| IBIS file k60_2m_180mhz_144mapbga_13x13_xn73j_derated.ibs generated by Viper version: 2018.10.16
[IBIS Ver]   4.2
[Comment Char]   |_char
[File Name]   k60_2m_180mhz_144mapbga_13x13_xn73j_derated.ibs
[File Rev]   1.0
[Date]   Tue Oct 16 17:54:02 2018
[Source]   NXP Viper 2018.10.16
[Notes]
[Disclaimer] IMPORTANT NOTICE
  This information is provided on an AS IS basis and without warranty.
  IN NO EVENT SHALL NXP BE LIABLE FOR INCIDENTAL OR CONSEQUENTIAL
  DAMAGES ARISING FROM USE OF THIS INFORMATION. THIS DISCLAIMER OF
  WARRANTY EXTENDS TO THE USER OF THE INFORMATION, AND TO THEIR CUSTOMERS
  OR USERS OF PRODUCTS  AND IS IN LIEU OF ALL WARRANTIES WHETHER EXPRESS,
  IMPLIED, OR STATUTORY, INCLUDING IMPLIED WARRANTIES OF MERCHANTABILITY
  OR FITNESS FOR PARTICULAR PURPOSE.
  NXP does not represent or warrant that the information furnished
  hereunder is free of infringement of any third party patents,
  copyrights, trade secrets, or other intellectual property rights.
  NXP does not represent or warrant that the information is free of
  defect, or that it meets any particular standard, requirements or need
  of the user of the infomation or their customers.
  NXP reserves the right to change the information in this file
  without notice.
   http://www.nxp.com
[Copyright]   (C) Copyright NXP 2004 - 2018, All Rights Reserved.
|   k60_2m_144mapbga_13x13
[Component]   k60_2m_144mapbga_13x13
[Manufacturer]   NXP
[Package]
| variable   typ   min   max
R_pkg   0.13037   0.042059   0.28237
L_pkg   2.200e-09   1.007e-09   4.756e-09
C_pkg   1.108e-12   8.202e-13   2.263e-12
[Pin] signal_name   model_name   R_pin   L_pin   C_pin
A1   PTD7   p_io_fast_hd_84u3v_6m   0.1767   3.230e-09 1.380e-12
A2   PTD6   p_io_fast_hd_84u3v_6m   0.24124   3.607e-09 1.256e-12
A3   PTD5   p_io_fast_hd_84u3v_6m   0.20685   3.225e-09 1.178e-12
A4   PTD4   p_io_fast_hd_84u3v_6m   0.1989   3.110e-09 1.168e-12
A5   PTD0   p_io_fast_84u3v_6m   0.16563   2.686e-09 1.012e-12
A6   PTC16   p_io_fast_84u3v_6m   0.16815   2.638e-09 1.005e-12
A7   PTC12   p_io_fast_84u3v_6m   0.15584   2.576e-09 1.008e-12
A8   PTC8   p_io_fast_84u3v_6m   0.15772   2.632e-09 9.509e-13
A9   PTC4   p_io_fast_hd_84u3v_6m   0.12744   2.310e-09 9.538e-13
A11   PTC3   p_io_fast_hd_84u3v_6m   0.17723   2.897e-09 1.109e-12
A12   PTC2   p_io_fast_84u3v_6m   0.20689   3.392e-09 1.147e-12
B1   PTD12   p_io_fast_84u3v_6m   0.20681   3.347e-09 1.070e-12
B2   PTD11   p_io_fast_84u3v_6m   0.15374   2.624e-09 1.135e-12
B3   PTD10   p_io_fast_84u3v_6m   0.14183   2.420e-09 1.169e-12
B4   PTD3   p_io_fast_84u3v_6m   0.15752   2.572e-09 1.158e-12
B5   PTC19   p_io_fast_84u3v_6m   0.14305   2.368e-09 9.679e-13
B6   PTC15   p_io_fast_84u3v_6m   0.18186   2.838e-09 1.206e-12
B7   PTC11   p_io_fast_84u3v_6m   0.1211   2.128e-09 1.062e-12
B8   PTC7   p_io_fast_84u3v_6m   0.115   2.073e-09 9.642e-13
B9   PTD9   p_io_fast_84u3v_6m   0.28237   4.756e-09 2.263e-12
B11   PTC1   p_io_fast_84u3v_6m   0.15165   2.581e-09 1.116e-12
B12   PTC0   p_io_fast_84u3v_6m   0.17659   2.976e-09 1.058e-12
C1   PTD15   p_io_fast_84u3v_6m   0.1459   2.559e-09 1.032e-12
C2   PTD14   p_io_fast_84u3v_6m   0.11803   2.152e-09 9.752e-13
C3   PTD13   p_io_fast_84u3v_6m   0.10442   1.941e-09 1.039e-12
C4   PTD2   p_io_fast_84u3v_6m   0.1542   2.591e-09 1.174e-12
C5   PTC18   p_io_fast_84u3v_6m   0.13918   2.329e-09 1.232e-12
C6   PTC14   p_io_fast_84u3v_6m   0.14045   2.324e-09 1.243e-12
C7   PTC10   p_io_fast_84u3v_6m   0.091438  1.815e-09 1.163e-12
C8   PTC6   p_io_fast_84u3v_6m   0.095955  1.862e-09 1.095e-12
C9   PTD8   p_io_fast_84u3v_6m   0.17703   3.145e-09 1.523e-12
C11   PTB23   p_io_fast_84u3v_6m   0.12401   2.224e-09 1.010e-12
C12   PTB22   p_io_fast_84u3v_6m   0.16109   2.737e-09 1.000e-12
D1   PTE2   p_io_fast_84u3v_6m   0.15458   2.571e-09 9.707e-13
D2   PTE1   p_io_fast_84u3v_6m   0.084672  1.697e-09 9.052e-13
D3   PTE0   p_io_fast_84u3v_6m   0.080898  1.614e-09 9.614e-13
D4   PTD1   p_io_fast_84u3v_6m   0.1196   2.013e-09 1.284e-12
D5   PTC17   p_io_fast_84u3v_6m   0.11589   1.937e-09 1.329e-12
D6   PTC13   p_io_fast_84u3v_6m   0.12216   2.016e-09 1.294e-12
D7   PTC9   p_io_fast_84u3v_6m   0.10769   1.891e-09 1.275e-12
D8   PTC5   p_io_fast_84u3v_6m   0.083046  1.529e-09 1.075e-12
D9   PTB21   p_io_fast_84u3v_6m   0.069786  1.388e-09 1.081e-12
D10   PTB20   p_io_fast_84u3v_6m   0.072983  1.512e-09 1.080e-12
D11   PTB19   p_io_fast_84u3v_6m   0.11729   2.101e-09 1.049e-12
D12   PTB18   p_io_fast_84u3v_6m   0.15379   2.582e-09 9.778e-13
E1   PTE6   p_io_fast_84u3v_6m   0.15201   2.497e-09 9.728e-13
E2   PTE5   p_io_fast_84u3v_6m   0.072065  1.467e-09 9.777e-13
E3   PTE4   p_io_fast_84u3v_6m   0.15445   2.567e-09 1.210e-12
E4   PTE3   p_io_fast_84u3v_6m   0.091528  1.512e-09 1.079e-12
E5   VDD   POWER   NA   NA   NA
E6   VDD   POWER   NA   NA   NA
E7   VDD   POWER   NA   NA   NA
E8   VDD   POWER   NA   NA   NA
E9   PTB17   p_io_fast_84u3v_6m   0.090018  1.530e-09 1.105e-12
E10   PTB16   p_io_fast_84u3v_6m   0.071785  1.356e-09 1.033e-12
E11   PTB11   p_io_fast_84u3v_6m   0.1174   2.042e-09 9.782e-13
E12   PTB10   p_io_fast_84u3v_6m   0.14971   2.513e-09 1.021e-12
F1   PTE10   p_io_fast_84u3v_6m   0.1489   2.421e-09 9.276e-13
F2   PTE9   p_io_fast_84u3v_6m   0.11513   1.993e-09 1.042e-12
F3   PTE8   p_io_fast_84u3v_6m   0.15002   2.498e-09 1.179e-12
F4   PTE7   p_io_fast_84u3v_6m   0.086683  1.500e-09 1.160e-12
F5   VDD   POWER   NA   NA   NA
F6   VSS   GND   NA   NA   NA
F7   VSS   GND   NA   NA   NA
F8   VDD   POWER   NA   NA   NA
F9   PTB9   p_io_fast_84u3v_6m   0.059202  1.173e-09 1.018e-12
F10   PTB8   p_io_fast_84u3v_6m   0.070195  1.393e-09 9.710e-13
F11   PTB7   p_io_fast_84u3v_6m   0.10803   1.929e-09 9.562e-13
F12   PTB6   p_io_fast_84u3v_6m   0.14447   2.427e-09 9.618e-13
G1   VREGOUT   POWER   0.063206  1.451e-09 1.324e-12
G2   VREGIN0   POWER   0.042059  1.007e-09 1.354e-12
G3   PTE12   p_io_fast_84u3v_6m   0.075407  1.340e-09 1.180e-12
G4   PTE11   p_io_fast_84u3v_6m   0.080602  1.557e-09 1.230e-12
G5   VREFH   POWER   NA   NA   NA
G6   VREFL   NC   NA   NA   NA
G7   VSS   GND   NA   NA   NA
G8   VSS   GND   NA   NA   NA
G9   PTB5   p_io_fast_84u3v_6m   0.08967   1.495e-09 1.046e-12
G10   PTB4   p_io_fast_84u3v_6m   0.067218  1.294e-09 9.258e-13
G11   PTB3   p_io_fast_84u3v_6m   0.11289   1.909e-09 9.538e-13
G12   PTB2   p_io_fast_84u3v_6m   0.15155   2.485e-09 9.892e-13
H1   USB0DP   NC   0.17782   2.688e-09 1.062e-12
H2   USB0DM   NC   0.16924   2.555e-09 1.175e-12
H3   VSS   GND   NA   NA   NA
H4   PTE28   p_io_fast_84u3v_6m   0.13628   2.231e-09 1.535e-12
H5   VDDA   POWER   NA   NA   NA
H6   VSSA   GND   NA   NA   NA
H7   VSS   GND   NA   NA   NA
H8   VSS   GND   NA   NA   NA
H9   PTB1   p_io_fast_hd_84u3v_6m   0.088545  1.541e-09 1.078e-12
H10   PTB0   p_io_fast_hd_84u3v_6m   0.07193   1.458e-09 1.011e-12
H11   PTA29   p_io_fast_84u3v_6m   0.1092   1.928e-09 9.740e-13
H12   PTA28   p_io_fast_84u3v_6m   0.1489   2.462e-09 9.911e-13
J1   USB1DP   NC   0.15803   2.269e-09 9.367e-13
J2   VREGIN1   POWER   0.068056  1.347e-09 1.170e-12
J3   ADC0SE16_CMP1IN2_ADC0SE21   NC   0.08836   1.703e-09 1.177e-12
J4   PTE27   p_io_fast_84u3v_6m   0.13178   2.323e-09 1.598e-12
J5   PTA0   p_io_fast_84u3v_6m   0.153   2.517e-09 1.320e-12
J6   PTA1   p_io_fast_84u3v_6m   0.13311   2.225e-09 1.256e-12
J7   PTA6   p_io_fast_84u3v_6m   0.062001  1.109e-09 1.055e-12
J8   PTA7   p_io_fast_84u3v_6m   0.084534  1.447e-09 1.157e-12
J9   PTA13   p_io_fast_84u3v_6m   0.07581   1.411e-09 1.087e-12
J10   PTA27   p_io_fast_84u3v_6m   0.062053  1.319e-09 1.092e-12
J11   PTA26   p_io_fast_84u3v_6m   0.109   1.945e-09 9.549e-13
J12   PTA25   p_io_fast_84u3v_6m   0.14712   2.455e-09 9.664e-13
K1   USB1DM   NC   0.15596   2.273e-09 9.297e-13
K2   VSS   GND   NA   NA   NA
K3   ADC1SE16_CMP2IN2_ADC0SE22   NC   0.093833  1.575e-09 9.911e-13
K4   PTE26   p_io_fast_84u3v_6m   0.11535   2.135e-09 1.578e-12
K5   PTE25   p_io_fast_84u3v_6m   0.071914  1.400e-09 1.592e-12
K6   PTA2   p_io_fast_84u3v_6m   0.075006  1.515e-09 1.067e-12
K7   PTA3   p_io_fast_84u3v_6m   0.076031  1.521e-09 9.091e-13
K8   PTA8   p_io_fast_84u3v_6m   0.16395   2.596e-09 1.171e-12
K9   PTA12   p_io_fast_84u3v_6m   0.077963  1.574e-09 1.040e-12
K10   PTA16   p_io_fast_84u3v_6m   0.12551   2.032e-09 1.168e-12
K11   PTA17   p_io_fast_84u3v_6m   0.14656   2.272e-09 1.166e-12
K12   PTA24   p_io_fast_84u3v_6m   0.12128   2.134e-09 9.407e-13
L1   USB1VBUS   POWER   0.090888  1.827e-09 1.559e-12
L2   ADC0DM0_ADC1DM3   NC   0.18325   2.692e-09 1.086e-12
L3   DAC0OUT_CMP1IN3_ADC0SE23   NC   0.11875   2.000e-09 8.994e-13
L4   DAC1OUT_CMP0IN4_CMP2IN3_ADC1SE23   NC   0.11014   1.898e-09 9.220e-13
L5   TAMPER0   p_io_84u3v_6m   0.12121   2.052e-09 1.037e-12
L6   VBAT   POWER   NA   NA   NA
L7   PTA4   p_io_flt_84u3v_6m   0.11174   1.932e-09 9.675e-13
L8   PTA9   p_io_fast_84u3v_6m   0.11121   1.866e-09 9.390e-13
L9   PTA11   p_io_fast_84u3v_6m   0.12511   2.024e-09 1.052e-12
L10   PTA14   p_io_fast_84u3v_6m   0.14162   2.139e-09 1.035e-12
L11   PTA15   p_io_fast_84u3v_6m   0.15537   2.405e-09 1.085e-12
L12   RESETB   p_vpp_84u3v_6m   0.12232   2.220e-09 1.068e-12
M1   ADC1DP0_ADC0DP3   NC   0.22009   3.293e-09 1.235e-12
M2   ADC1DM0_ADC0DM3   NC   0.22652   3.293e-09 1.206e-12
M3   VREFOUT_CMP1IN5_CMP0IN5_ADC1SE18   NC   0.17041   2.710e-09 9.453e-13
M4   PTE24   p_io_fast_84u3v_6m   0.18414   2.868e-09 1.024e-12
M6   EXTAL32   NC   0.13257   2.260e-09 8.202e-13
M7   XTAL32   NC   0.18902   3.006e-09 1.031e-12
M8   PTA5   p_io_fast_84u3v_6m   0.1639   2.449e-09 1.034e-12
M9   PTA10   p_io_fast_84u3v_6m   0.16013   2.533e-09 1.014e-12
M10   VSS   GND   NA   NA   NA
M11   PTA19   p_io_fast_84u3v_6m   0.21862   3.056e-09 1.159e-12
M12   PTA18   p_io_fast_84u3v_6m   0.17651   2.672e-09 1.041e-12
[Pin Mapping]   pulldown_ref   pullup_ref
A1   NC   NC
A2   NC   NC
A3   NC   NC
A4   NC   NC
A5   NC   NC
A6   NC   NC
A7   NC   NC
A8   NC   NC
A9   NC   NC
A11   NC   NC
A12   NC   NC
B1   NC   NC
B2   NC   NC
B3   NC   NC
B4   NC   NC
B5   NC   NC
B6   NC   NC
B7   NC   NC
B8   NC   NC
B9   NC   NC
B11   NC   NC
B12   NC   NC
C1   NC   NC
C2   NC   NC
C3   NC   NC
C4   NC   NC
C5   NC   NC
C6   NC   NC
C7   NC   NC
C8   NC   NC
C9   NC   NC
C11   NC   NC
C12   NC   NC
D1   NC   NC
D2   NC   NC
D3   NC   NC
D4   NC   NC
D5   NC   NC
D6   NC   NC
D7   NC   NC
D8   NC   NC
D9   NC   NC
D10   NC   NC
D11   NC   NC
D12   NC   NC
E1   NC   NC
E2   NC   NC
E3   NC   NC
E4   NC   NC
E5   NC   VDD
E6   NC   VDD
E7   NC   VDD
E8   NC   VDD
E9   NC   NC
E10   NC   NC
E11   NC   NC
E12   NC   NC
F1   NC   NC
F2   NC   NC
F3   NC   NC
F4   NC   NC
F5   NC   VDD
F6   VSS   NC
F7   VSS   NC
F8   NC   VDD
F9   NC   NC
F10   NC   NC
F11   NC   NC
F12   NC   NC
G1   NC   VREGOUT
G2   NC   VREGIN0
G3   NC   NC
G4   NC   NC
G5   NC   VREFH
G6   NC   NC
G7   VSS   NC
G8   VSS   NC
G9   NC   NC
G10   NC   NC
G11   NC   NC
G12   NC   NC
H1   NC   NC
H2   NC   NC
H3   VSS   NC
H4   NC   NC
H5   NC   VDDA
H6   VSSA   NC
H7   VSS   NC
H8   VSS   NC
H9   NC   NC
H10   NC   NC
H11   NC   NC
H12   NC   NC
J1   NC   NC
J2   NC   VREGIN1
J3   NC   NC
J4   NC   NC
J5   NC   NC
J6   NC   NC
J7   NC   NC
J8   NC   NC
J9   NC   NC
J10   NC   NC
J11   NC   NC
J12   NC   NC
K1   NC   NC
K2   VSS   NC
K3   NC   NC
K4   NC   NC
K5   NC   NC
K6   NC   NC
K7   NC   NC
K8   NC   NC
K9   NC   NC
K10   NC   NC
K11   NC   NC
K12   NC   NC
L1   NC   USB1VBUS
L2   NC   NC
L3   NC   NC
L4   NC   NC
L5   NC   NC
L6   NC   VBAT
L7   NC   NC
L8   NC   NC
L9   NC   NC
L10   NC   NC
L11   NC   NC
L12   NC   NC
M1   NC   NC
M2   NC   NC
M3   NC   NC
M4   NC   NC
M6   NC   NC
M7   NC   NC
M8   NC   NC
M9   NC   NC
M10   VSS   NC
M11   NC   NC
M12   NC   NC
|*   Model Selector   *
[Model Selector] p_io_84u3v_6m
p_io_84u3v_6m_sre0   io, without slew rate
p_io_84u3v_6m_sre1   io, with slew rate
[Model Selector] p_io_fast_84u3v_6m
p_io_fast_84u3v_6m_sre0   io, without slew rate
p_io_fast_84u3v_6m_sre1   io, with slew rate
[Model Selector] p_io_fast_hd_84u3v_6m
p_io_fast_hd_84u3v_6m_obe1dse0sre0   io 5mA, without slew rate
p_io_fast_hd_84u3v_6m_obe1dse0sre1   io 5mA, with slew rate
p_io_fast_hd_84u3v_6m_obe1dse1sre0   io 20mA, without slew rate
p_io_fast_hd_84u3v_6m_obe1dse1sre1   io 20mA, with slew rate
[Model Selector] p_io_flt_84u3v_6m
p_io_flt_84u3v_6m_sre0   io_flt, without slew rate
p_io_flt_84u3v_6m_sre1   io_flt, with slew rate
| End [Component] k60_2m_144mapbga_13x13
| Models and submodels in the file (11): p_io_84u3v_6m_sre0 (I/O), p_io_84u3v_6m_sre1 (I/O), p_io_fast_84u3v_6m_sre0 (I/O), p_io_fast_84u3v_6m_sre1 (I/O), p_io_fast_hd_84u3v_6m_obe1dse0sre0 (I/O), p_io_fast_hd_84u3v_6m_obe1dse0sre1 (I/O), p_io_fast_hd_84u3v_6m_obe1dse1sre0 (I/O), p_io_fast_hd_84u3v_6m_obe1dse1sre1 (I/O), p_io_flt_84u3v_6m_sre0 (I/O), p_io_flt_84u3v_6m_sre1 (I/O), p_vpp_84u3v_6m (I/O_open_drain)
